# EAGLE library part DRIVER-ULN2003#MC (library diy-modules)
7-Channel Darlington NPN Transistor Module based on ULN2003 chip Symbol with motor connector pins More details available here: https://www.elecrow.com/wiki/index.php?title=ULN2003_Stepper_Motor_Driver ULN2003 datasheet available here: http://www.ti.com/lit/ds/slrs027o/slrs027o.pdf Click here to find device on ebay.com Note: There are many variants. Search for the proper version.
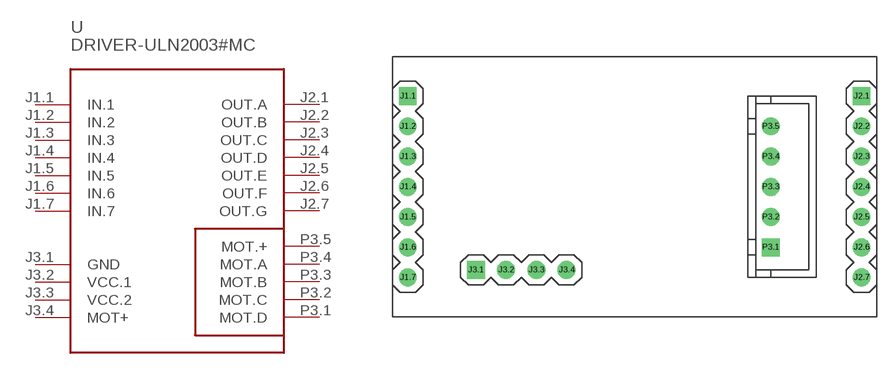
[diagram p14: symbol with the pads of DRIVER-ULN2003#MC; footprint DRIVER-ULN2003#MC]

Designator prefix -

## DRIVER-ULN2003#MC  [DRIVER-ULN2003#MC]
J1.1  IN.1
J1.2  IN.2
J1.3  IN.3
J1.4  IN.4
J1.5  IN.5
J1.6  IN.6
J1.7  IN.7
J2.1  OUT.A
J2.2  OUT.B
J2.3  OUT.C
J2.4  OUT.D
J2.5  OUT.E
J2.6  OUT.F
J2.7  OUT.G
J3.1  GND  pwr
J3.2  VCC.1  pwr
J3.3  VCC.2
J3.4  MOT+
P3.1  MOT.D
P3.2  MOT.C
P3.3  MOT.B
P3.4  MOT.A
P3.5  MOT.+

## Footprint DRIVER-ULN2003#MC (pad centres in mm)
7-Channel Darlington NPN Transistor Module based on ULN2003 chip Footprint with motor connector
drill 1 square: J1.1 -19.05,7.62; J2.1 19.05,7.62; J3.1 -13.335,-6.985; P3.1 11.43,-5.08
drill 1: J1.2 -19.05,5.08; J1.3 -19.05,2.54; J1.4 -19.05,0; J1.5 -19.05,-2.54; J1.6 -19.05,-5.08; J1.7 -19.05,-7.62; J2.2 19.05,5.08; J2.3 19.05,2.54; J2.4 19.05,0; J2.5 19.05,-2.54; J2.6 19.05,-5.08; J2.7 19.05,-7.62; J3.2 -10.795,-6.985; J3.3 -8.255,-6.985; J3.4 -5.715,-6.985; P3.2 11.43,-2.54; P3.3 11.43,0; P3.4 11.43,2.54; P3.5 11.43,5.08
